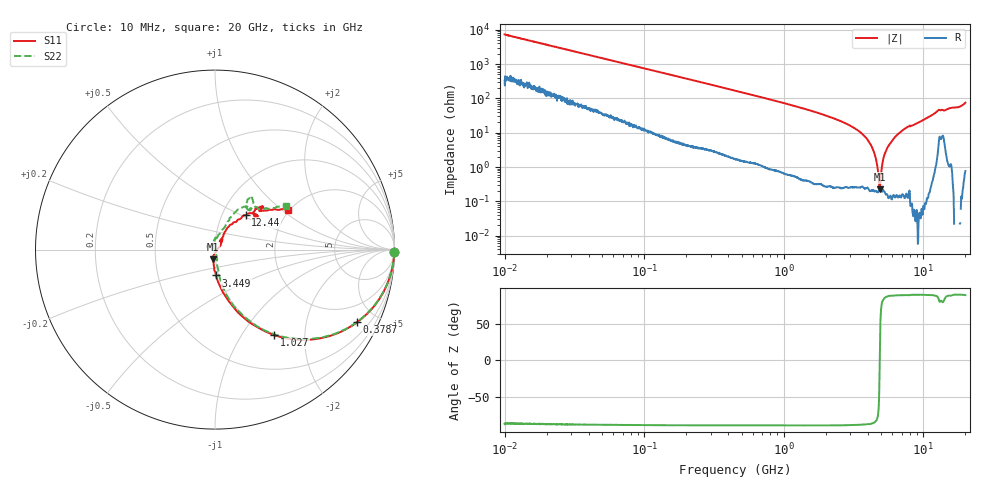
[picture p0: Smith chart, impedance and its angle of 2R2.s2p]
!Keysight Technologies,P5008B,MY61100088,A.16.20.02
!Date: Friday, August 30, 2024 11:13:47
!Correction: S11(C  2-Port  )
!S21(C  2-Port  )
!S12(C  2-Port  )
!S22(C  2-Port  )
!S2P File: Measurements: S11, S21, S12, S22:Log Frequency Sweep
# Hz S  dB  R 50
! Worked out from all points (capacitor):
!   1601 points, 10 MHz to 20 GHz, reference 50 ohm
!   read as one part in series: C = 2.2 pF near 10.39 MHz
!   lowest |Z| = 227 mohm at 4.855 GHz (marker M1)
!   series resonance near 4.866 GHz, so ESL is about 490 pH
!   S11 on the Smith chart (normalised r, x): 10 MHz: open; 378.7 MHz: 1.01, -3.91; 1.027 GHz: 0.98, -1.41; 3.449 GHz: 0.97, -0.29; 12.44 GHz: 1.29, +0.53; 20 GHz: 1.95, +1.11
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1e7  -0.00 -0.8  -37.20 86.6  -37.19 86.5  -0.01 -0.8
3.555162e7  -0.02 -2.8  -26.33 85.5  -26.34 85.5  -0.02 -2.8
1.263918e8  -0.14 -9.7  -15.60 79.5  -15.61 79.5  -0.14 -9.6
3.787084e8  -1.02 -27.0  -6.99 62.5  -6.99 62.5  -1.02 -26.8
4.472136e8  -1.36 -31.2  -5.87 58.4  -5.88 58.4  -1.35 -30.9
1.026987e9  -4.72 -55.2  -1.84 34.6  -1.85 34.6  -4.72 -54.7
1.589917e9  -7.91 -67.8  -0.79 22.2  -0.80 22.2  -7.91 -66.8
3.44879e9  -16.83 -87.8  -0.11 4.4  -0.11 4.3  -16.73 -81.2
4.855267e9  -25.25 -102.6  -0.02 -3.0  -0.03 -3.0  -25.09 -77.2
5.652411e9  -31.53 -101.2  -0.00 -6.3  -0.01 -6.4  -32.04 -79.9
5.899321e9  -34.74 -92.4  0.01 -7.3  0.00 -7.3  -35.65 -83.5
6.098795e9  -37.41 -64.7  0.01 -8.0  0.00 -8.1  -41.08 -98.8
6.275133e9  -40.27 -21.2  0.01 -8.7  0.00 -8.7  -50.06 161.0
6.425969e9  -36.83 6.1  0.01 -9.2  0.01 -9.3  -41.18 123.4
6.770695e9  -31.38 29.5  0.01 -10.5  0.01 -10.5  -32.71 111.7
7.410252e9  -26.09 47.1  0.01 -12.8  0.00 -12.8  -26.53 98.1
7.697294e9  -24.54 56.0  0.00 -13.7  -0.00 -13.8  -24.89 88.8
8.750704e9  -24.46 60.9  0.01 -17.2  0.01 -17.3  -24.42 78.9
1.2437e10  -11.77 48.4  -0.35 -31.6  -0.36 -31.7  -11.79 60.3
1.387292e10  -10.69 37.4  -0.92 -31.8  -0.92 -31.9  -10.64 48.0
1.717946e10  -9.29 41.6  -0.47 -43.4  -0.48 -43.6  -9.34 51.2
2e10  -6.67 28.7  -1.07 -58.7  -1.07 -58.9  -6.60 31.7
